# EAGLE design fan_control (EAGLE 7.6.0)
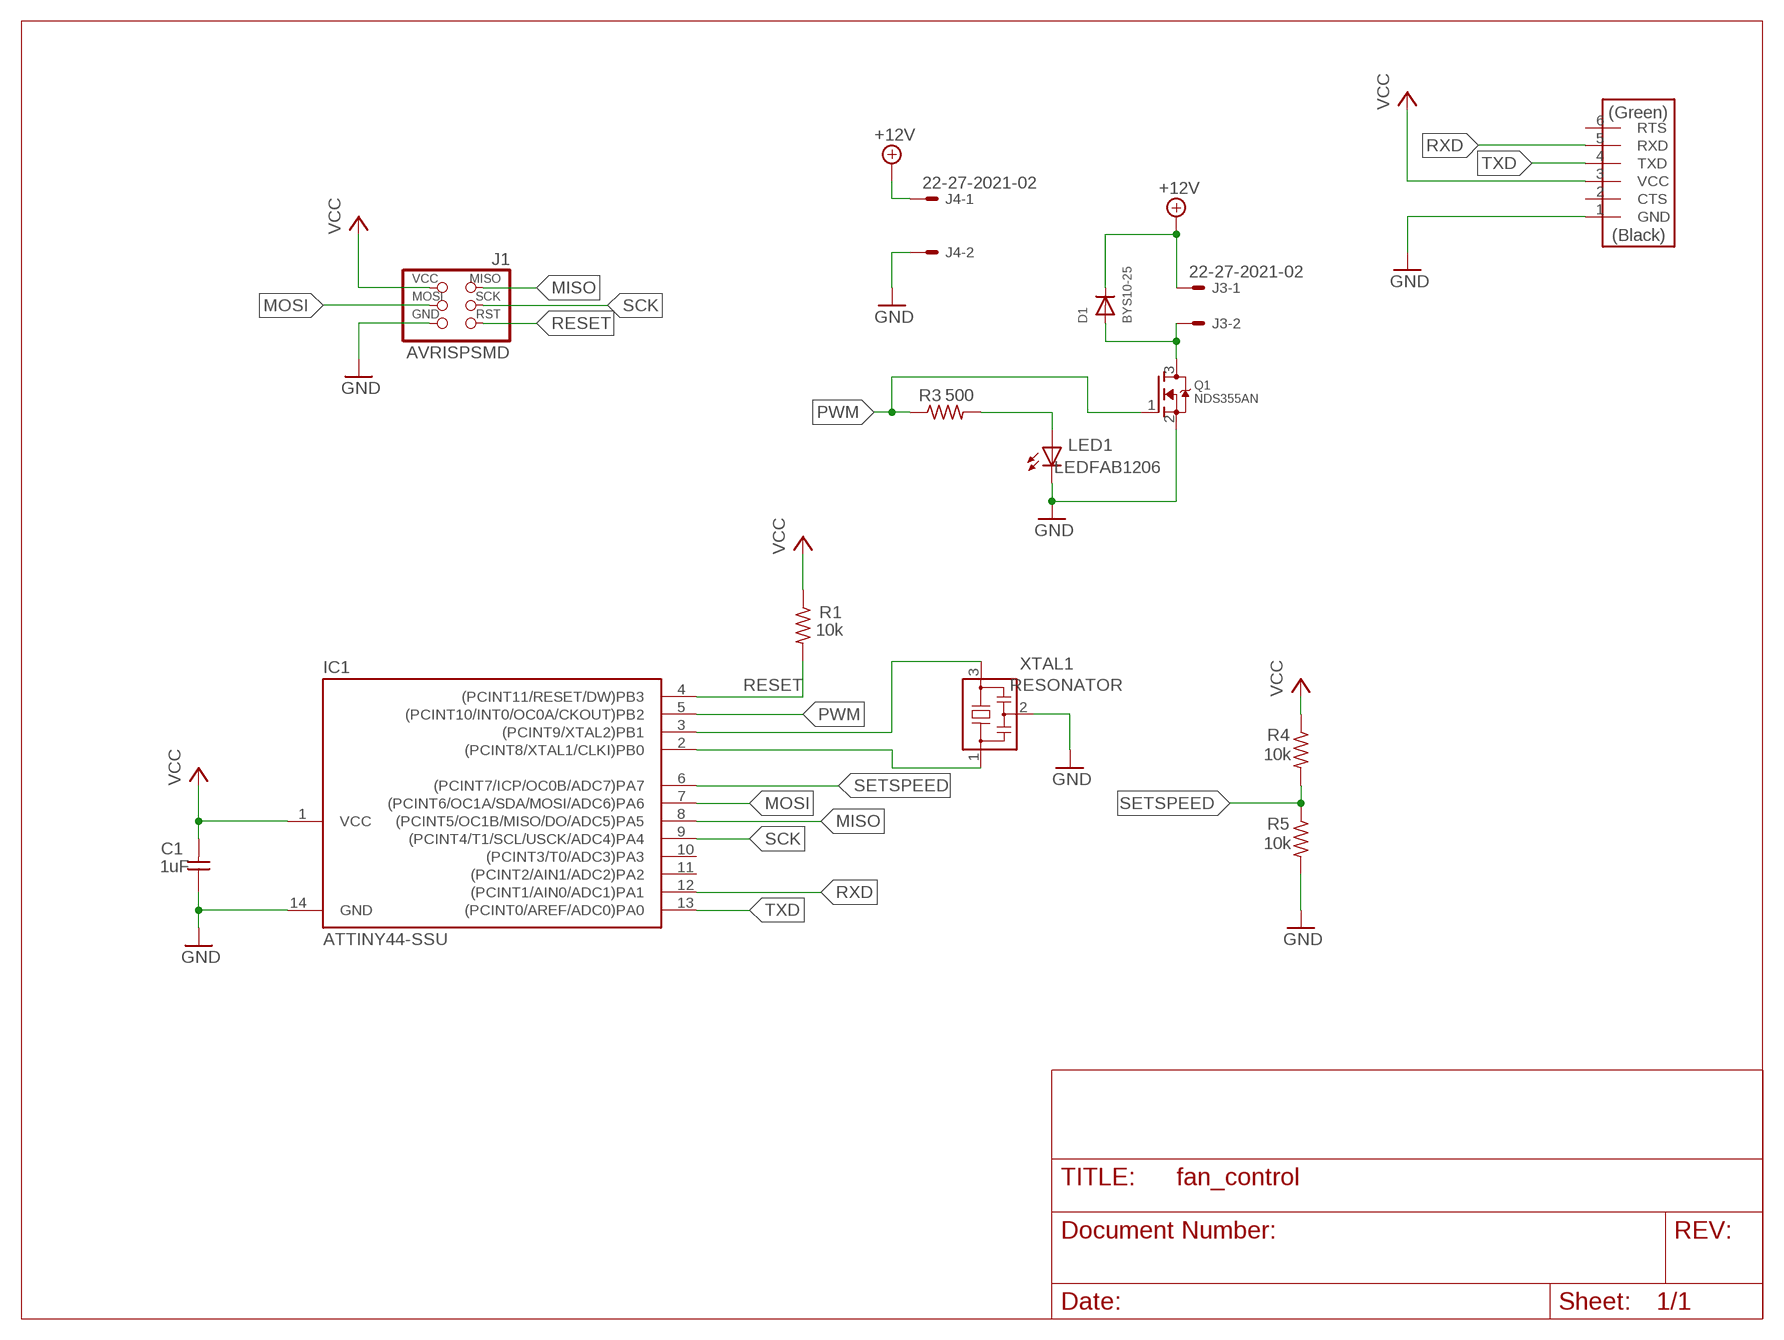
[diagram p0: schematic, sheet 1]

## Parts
C1  1uF  CAP-UNPOLARIZEDFAB  [C1206FAB]
D1  BYS10-25  DIODESMA  [SMADIODE]
IC1  ATTINY44-SSU  [SOIC14]
J1  AVRISPSMD  [2X03SMD]
J2  FTDI-SMD-HEADER  [1X06SMD]
J3  22-27-2021-02  [6410-02]
J4  22-27-2021-02  [6410-02]
LED1  LEDFAB1206  [LED1206FAB]
Q1  NDS355AN  MOSFET-NREFLOW  [SOT23]
R1  10k  RES-US1206FAB  [R1206FAB]
R3  500  RES-US1206FAB  [R1206FAB]
R4  10k  RES-US1206FAB  [R1206FAB]
R5  10k  RES-US1206FAB  [R1206FAB]
XTAL1  RESONATOR  [EFOBM]

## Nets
+12V: D1.C J3.1 J4.1
GND: C1.1 IC1.14(GND) J1.6(GND) J2.1(GND) J4.2 LED1.2(C) Q1.2(S) R5.2 XTAL1.2
MISO: IC1.8((PCINT5/OC1B/MISO/DO/ADC5)PA5) J1.1(MISO)
MOSI: IC1.7((PCINT6/OC1A/SDA/MOSI/ADC6)PA6) J1.4(MOSI)
N$1: LED1.1(A) R3.2
N$2: IC1.3((PCINT9/XTAL2)PB1) XTAL1.3
N$3: D1.A J3.2 Q1.3(D)
PWM: IC1.5((PCINT10/INT0/OC0A/CKOUT)PB2) Q1.1(G) R3.1
RESET: IC1.4((PCINT11/RESET/DW)PB3) J1.5(RST) R1.2
RXD: IC1.12((PCINT1/AIN0/ADC1)PA1) J2.5(RXD)
SCK: IC1.9((PCINT4/T1/SCL/USCK/ADC4)PA4) J1.3(SCK)
SETSPEED: IC1.6((PCINT7/ICP/OC0B/ADC7)PA7) R4.2 R5.1
TXD: IC1.13((PCINT0/AREF/ADC0)PA0) J2.4(TXD)
VCC: C1.2 IC1.1(VCC) J1.2(VCC) J2.3(VCC) R1.1 R4.1
XTAL1: IC1.2((PCINT8/XTAL1/CLKI)PB0) XTAL1.1
Unconnected: IC1.10((PCINT3/T0/ADC3)PA3) IC1.11((PCINT2/AIN1/ADC2)PA2) J2.2(CTS) J2.6(RTS)

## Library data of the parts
C1 = fab:CAP-UNPOLARIZED
D1 = adafruit:DIODE: Diode
IC1 = fab:ATTINY44
J1 = fab:AVRISP
J2 = fab:FTDI-SMD-HEADER
J3 J4 = con-molex:22-?-02: CONNECTOR; OC_FARNELL: unknown; OC_NEWARK: unknown
LED1 = fab:LED: LED
Q1 = adafruit:MOSFET-N: N-Channel Mosfet 2N7002E - 60V 260mA SOT23 [Digikey: 2N7002ET1GOSTR-ND] - REEL BSH103 - 30V 850mA SOT23 [Digikey: 568-5013-1-ND]
R1 R3-R5 = fab:RES-US: Resistor (US Symbol)
XTAL1 = fab:RESONATOR

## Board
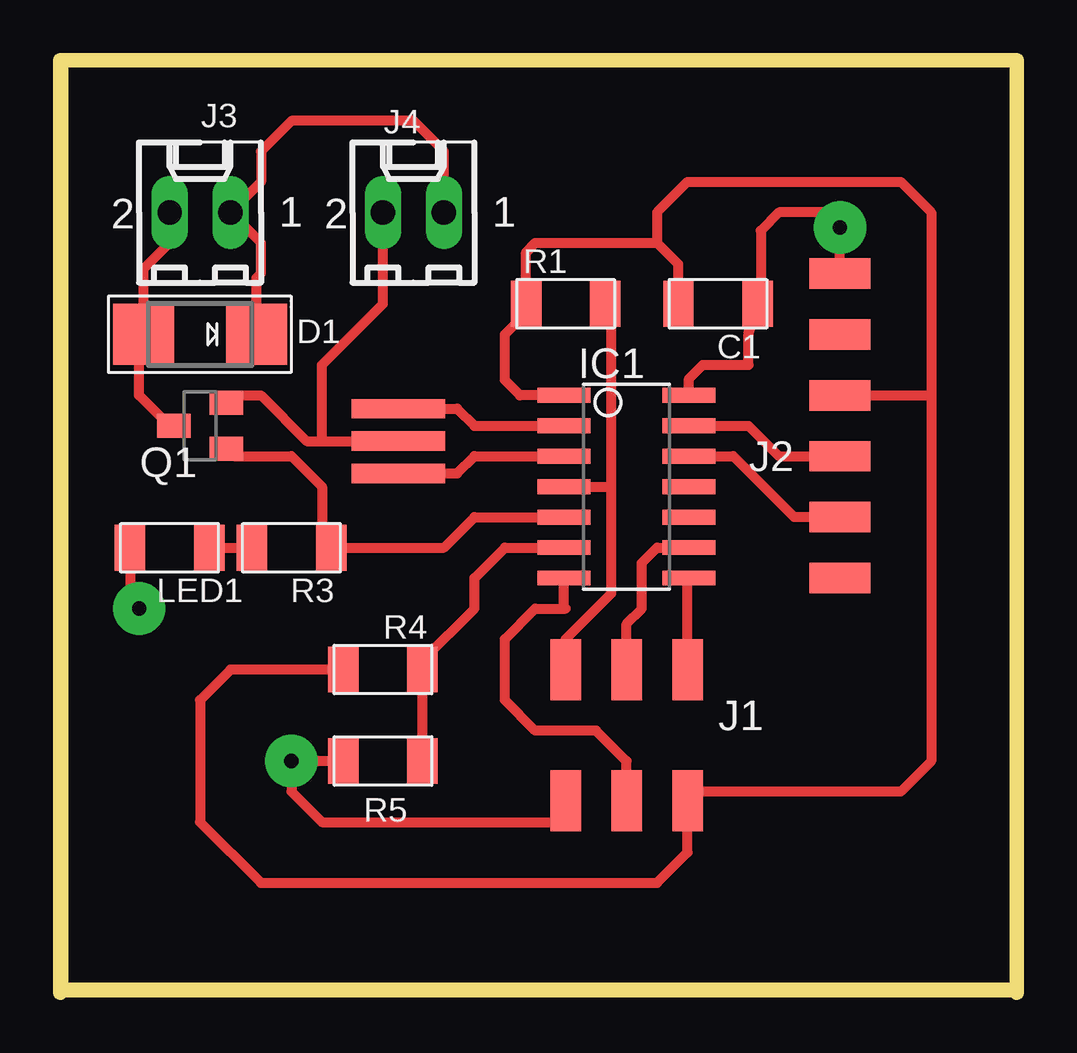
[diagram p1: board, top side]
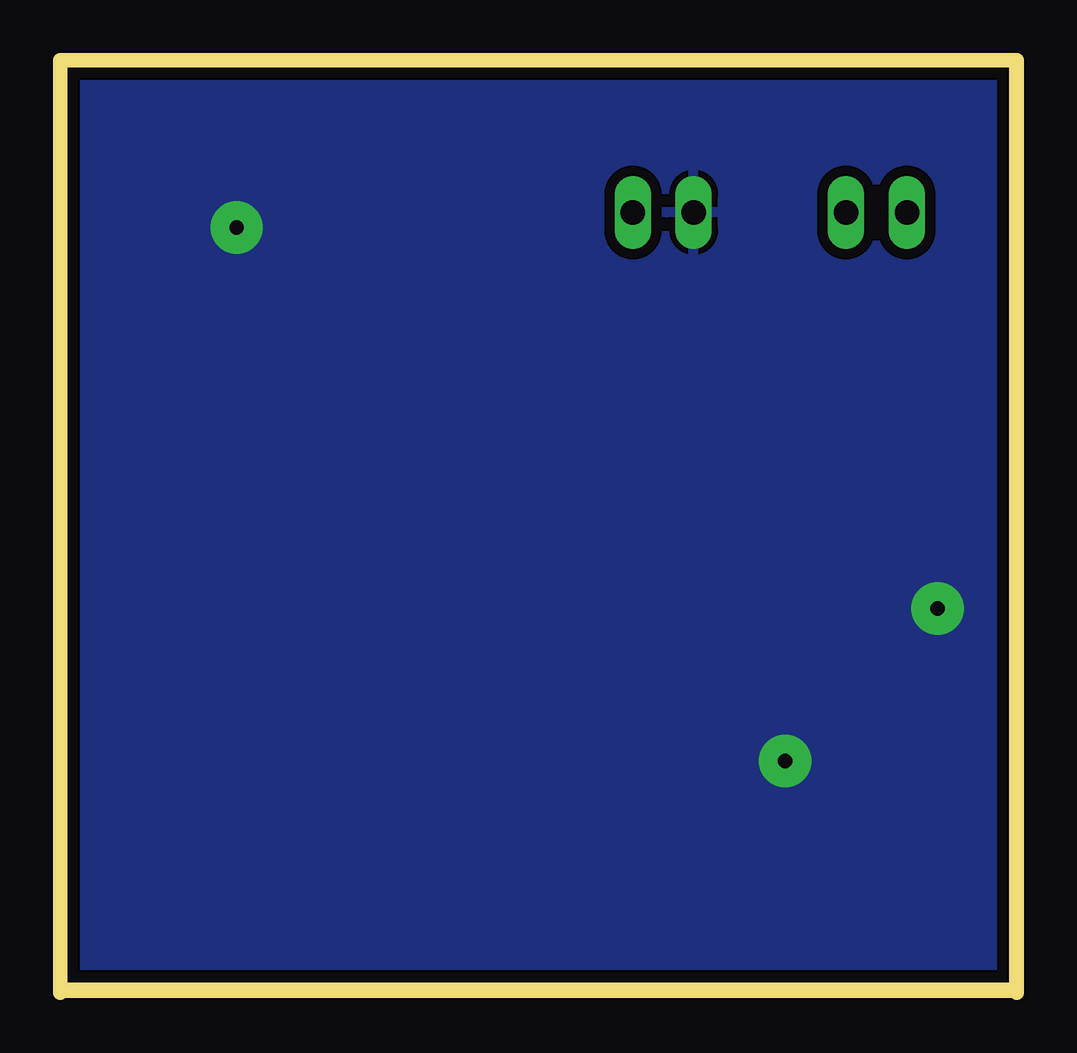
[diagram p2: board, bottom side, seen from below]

Size 39.88 x 38.86 mm. Coordinates in mm from the lower left corner, seen from the top.
Outline: 0.13,0.13 39.8,0.13 39.8,38.85 0.13,38.85 0.13,0.13
Outline: 0,38.86 39.88,38.86 39.88,0 0,0 0,38.86
Copper layers (1*16): Top 0.035mm / dielectric 1.5mm / Bottom 0.035mm
Design rules "default *": minimum track width 12mil, minimum drill 24mil, track to track 17mil, track to pad 16mil, pad to pad 16mil, via to via 16mil, smd to smd 8mil, copper to edge 20mil, drill to drill 8mil, minimum pad ring 10mil, minimum via ring 8mil, stop-mask expansion 4mil, vias tented up to drill 0mil, thermal gap 10mil

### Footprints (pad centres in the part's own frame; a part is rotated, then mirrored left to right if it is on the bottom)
C1206FAB = smd 1.27 x 1.905: 1 -1.651,0; 2 1.651,0
SMADIODE = smd 2.54 x 2.54: A 2.349,0; C -2.349,0
SOIC14 = smd 0.61 x 2.21: 1 -3.81,-2.603; 2 -2.54,-2.603; 3 -1.27,-2.603; 4 0,-2.603; 5 1.27,-2.603; 6 2.54,-2.603; 7 3.81,-2.603; 8 3.81,2.603; 9 2.54,2.603; 10 1.27,2.603; 11 0,2.603; 12 -1.27,2.603; 13 -2.54,2.603; 14 -3.81,2.603
2X03SMD = smd 2.54 x 1.27: 1 -2.54,2.54; 2 2.92,2.54; 3 -2.54,0; 4 2.92,0; 5 -2.54,-2.54; 6 2.92,-2.54
1X06SMD = smd 2.54 x 1.27: 1 0,6.35; 2 0,3.81; 3 0,1.27; 4 0,-1.27; 5 0,-3.81; 6 0,-6.35
6410-02 = drill 1.016 long: 1 1.27,0; 2 -1.27,0
LED1206FAB = smd 1.27 x 1.905: 1 -1.651,0; 2 1.651,0
SOT23 = smd 1 x 1.4: 1 -0.95,-1.1; 2 0.95,-1.1; 3 0,1.1
R1206FAB = smd 1.27 x 1.905: 1 -1.651,0; 2 1.651,0
EFOBM = smd 0.8 x 3.9: 1 -1.35,0; 2 0,0; 3 1.35,0

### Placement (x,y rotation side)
C1  27.43,28.7 180 top
D1  5.84,27.43 180 top
IC1  23.62,21.08 270 top
J1  23.62,10.92 270 top
J2  32.51,23.62 0 top
J3  5.84,32.51 0 top
J4  14.73,32.51 0 top
LED1  4.57,18.54 180 top
Q1  5.84,23.62 90 top
R1  21.08,28.7 0 top
R3  9.65,18.54 180 top
R4  13.46,13.46 0 top
R5  13.46,9.65 180 top
XTAL1  14.1,22.99 270 top

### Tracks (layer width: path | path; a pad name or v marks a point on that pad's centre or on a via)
+12V
  Top 0.406: J4.1 16,35.05 14.73,36.32 9.65,36.32 8.38,35.05 8.38,33.78 J3.1 8.38,31.24 8.38,29.97 8.19,29.78 D1.C
GND  (via drill 0.6 pad 2.18)
  Top 0.406: Q1.2 7.26,24.89 8.38,24.89 10.29,22.99 10.92,22.99 | 10.92,22.99 XTAL1.2 | LED1.2 2.92,16.38 v3.3,16 | 10.92,22.99 10.92,26.16 13.46,28.7 J4.2 | IC1.14 26.22,25.59 26.8,26.16 28.7,26.16 28.7,27.43 C1.1 | 28.7,28.32 C1.1 | C1.1 29.08,29.08 | R5.2 v9.65,9.65 9.65,8.38 10.92,7.11 21.08,7.11 J1.6 | J2.1 v32.51,31.88 32.51,32.51 29.97,32.51 29.21,31.75 29.21,28.83 C1.1
  pour Bottom: -0.51,40.13 41.4,40.13 41.4,-0.51 -0.51,-0.51
MISO
  Top 0.406: J1.1 26.16,17.21 IC1.8
MOSI
  Top 0.406: J1.4 23.62,9.65 22.35,10.92 19.81,10.92 18.54,12.19 18.54,14.73 19.81,16 21.08,16 21.02,16.07 IC1.7
N$1
  Top 0.406: LED1.1 R3.2
N$2
  Top 0.406: XTAL1.3 16.56,21.64 17.27,22.35 IC1.3
N$3
  Top 0.406: J3.2 4.57,31.24 3.49,30.16 D1.A 3.3,27.24 3.3,24.89 4.57,23.62 Q1.3
PWM
  Top 0.406: IC1.5 17.27,19.81 16,18.54 R3.1 10.92,18.92 10.92,21.08 9.65,22.35 7.26,22.35 Q1.1
RESET
  Top 0.406: J1.5 21.08,14.73 22.99,16.64 22.99,21.08 | IC1.4 22.99,21.08 | 22.99,21.08 22.99,28.07 22.73,28.32 R1.2
RXD
  Top 0.406: IC1.12 28.07,22.35 30.61,19.81 J2.5
SCK
  Top 0.406: J1.3 23.62,15.37 24.26,16 24.26,17.91 24.89,18.54 IC1.9
SETSPEED
  Top 0.406: IC1.6 18.54,18.54 17.27,17.27 17.27,16 15.11,13.84 R4.2 R5.1
TXD
  Top 0.406: IC1.13 28.7,23.62 29.97,22.35 J2.4
VCC
  Top 0.406: IC1.1 19.18,24.89 18.54,25.53 18.54,27.43 19.43,28.32 R1.1 19.43,30.86 19.81,31.24 24.89,31.24 | C1.2 25.78,30.35 24.89,31.24 | J2.3 36.32,24.89 | 24.89,31.24 24.89,32.51 26.16,33.78 35.05,33.78 36.32,32.51 36.32,24.89 | 36.32,24.89 36.32,9.65 35.05,8.38 26.54,8.38 J1.2 26.16,5.84 24.89,4.57 8.38,4.57 5.84,7.11 5.84,12.19 7.11,13.46 R4.1
XTAL1
  Top 0.406: XTAL1.1 16.56,24.34 17.27,23.62 IC1.2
